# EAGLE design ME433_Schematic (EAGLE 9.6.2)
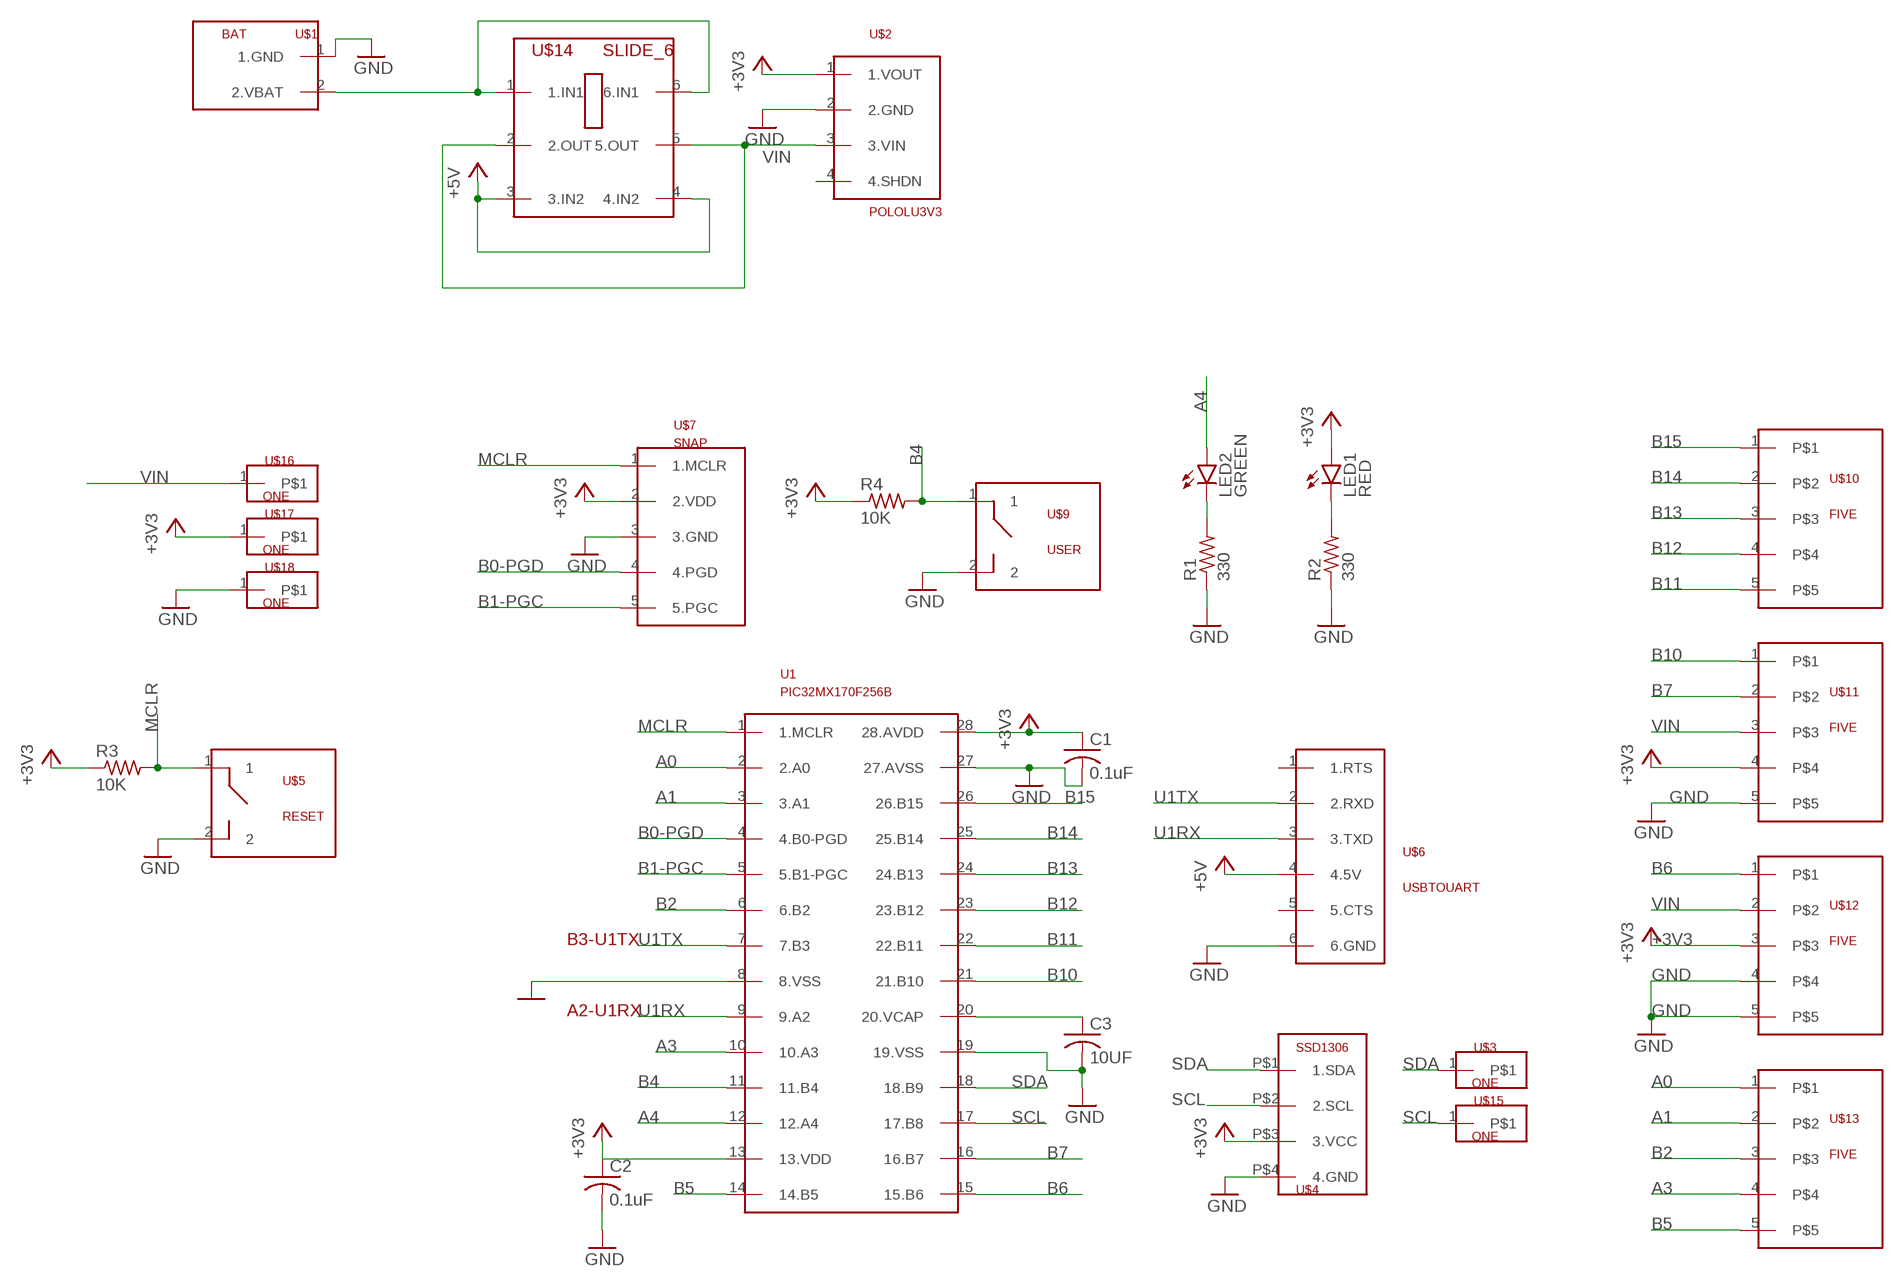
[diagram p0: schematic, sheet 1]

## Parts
C1  0.1uF  C-US025-030X050  [C025-030X050]
C2  0.1uF  C-US025-030X050  [C025-030X050]
C3  10UF  C-US025-030X050  [C025-030X050]
LED1  RED  LED3MM  [LED3MM]
LED2  GREEN  LED3MM  [LED3MM]
R1  330  R-US_0207/7  [0207/7]
R2  330  R-US_0207/7  [0207/7]
R3  10K  R-US_0207/7  [0207/7]
R4  10K  R-US_0207/7  [0207/7]
U1  PIC32MX170F256B  [DIL28-3]
U$1  BAT  [BAT]
U$2  POLOLU3V3  [POLOLU3V3]
U$3  ONE  [ONE]
U$4  SSD1306  [SSD1306]
U$5  RESET  BUTTON  [BUTTON]
U$6  USBTOUART  [USBTOUART]
U$7  SNAP  [SNAP]
U$9  USER  BUTTON  [BUTTON]
U$10  FIVE  [FIVE]
U$11  FIVE  [FIVE]
U$12  FIVE  [FIVE]
U$13  FIVE  [FIVE]
U$14  SLIDE_6  [SLIDE_6]
U$15  ONE  [ONE]
U$16  ONE  [ONE]
U$17  ONE  [ONE]
U$18  ONE  [ONE]

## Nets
+3V3: C1.1 C2.1 LED1.A R3.1 R4.1 U1.13(13.VDD) U1.28(28.AVDD) U$2.1(1.VOUT) U$4.P$3(3.VCC) U$7.2(2.VDD) U$11.4 U$12.3 U$17.1
+5V: U$6.4(4.5V) U$14.3(3.IN2) U$14.4(4.IN2)
A0: U1.2(2.A0) U$13.1
A1: U1.3(3.A1) U$13.2
A3: U1.10(10.A3) U$13.4
A4: LED2.A U1.12(12.A4)
B0-PGD: U1.4(4.B0-PGD) U$7.4(4.PGD)
B1-PGC: U1.5(5.B1-PGC) U$7.5(5.PGC)
B2: U1.6(6.B2) U$13.3
B4: R4.2 U1.11(11.B4) U$9.1
B5: U1.14(14.B5) U$13.5
B6: U1.15(15.B6) U$12.1
B7: U1.16(16.B7) U$11.2
B10: U1.21(21.B10) U$11.1
B11: U1.22(22.B11) U$10.5
B12: U1.23(23.B12) U$10.4
B13: U1.24(24.B13) U$10.3
B14: U1.25(25.B14) U$10.2
B15: U1.26(26.B15) U$10.1
GND: C1.2 C2.2 C3.2 R1.1 R2.1 U1.8(8.VSS) U1.19(19.VSS) U1.27(27.AVSS) U$1.1(1.GND) U$2.2(2.GND) U$4.P$4(4.GND) U$5.2 U$6.6(6.GND) U$7.3(3.GND) U$9.2 U$11.5 U$12.4 U$12.5 U$18.1
MCLR: R3.2 U1.1(1.MCLR) U$5.1 U$7.1(1.MCLR)
N$1: LED1.K(C) R2.2
N$2: LED2.K(C) R1.2
N$3: C3.1 U1.20(20.VCAP)
N$4: U$1.2(2.VBAT) U$14.1(1.IN1) U$14.6(6.IN1)
SCL: U1.17(17.B8) U$4.P$2(2.SCL) U$15.1
SDA: U1.18(18.B9) U$3.1 U$4.P$1(1.SDA)
U1RX: U1.9(9.A2) U$6.3(3.TXD)
U1TX: U1.7(7.B3) U$6.2(2.RXD)
VIN: U$2.3(3.VIN) U$11.3 U$12.2 U$14.2(2.OUT) U$14.5(5.OUT) U$16.1
Unconnected: U$2.4(4.SHDN) U$6.1(1.RTS) U$6.5(5.CTS)

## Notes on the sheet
- B3-U1TX
- A2-U1RX

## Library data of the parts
C1-C3 = ME433_Library:C-US: CAPACITOR, American symbol; SPICEPREFIX: C
LED1 LED2 = ME433_Library:LED: LED
R1-R4 = ME433_Library:R-US_: RESISTOR, American symbol; SPICEPREFIX: R
U1 = ME433_Library:PIC32MX170F256B
U$1 = ME433_Library:BAT
U$2 = ME433_Library:POLOLU3V3
U$3 U$15-U$18 = ME433_Library:ONE
U$4 = ME433_Library:SSD1306
U$5 U$9 = ME433_Library:BUTTON
U$6 = ME433_Library:USBTOUART
U$7 = ME433_Library:SNAP
U$10-U$13 = ME433_Library:FIVE
U$14 = ME433_Library:SLIDE_6

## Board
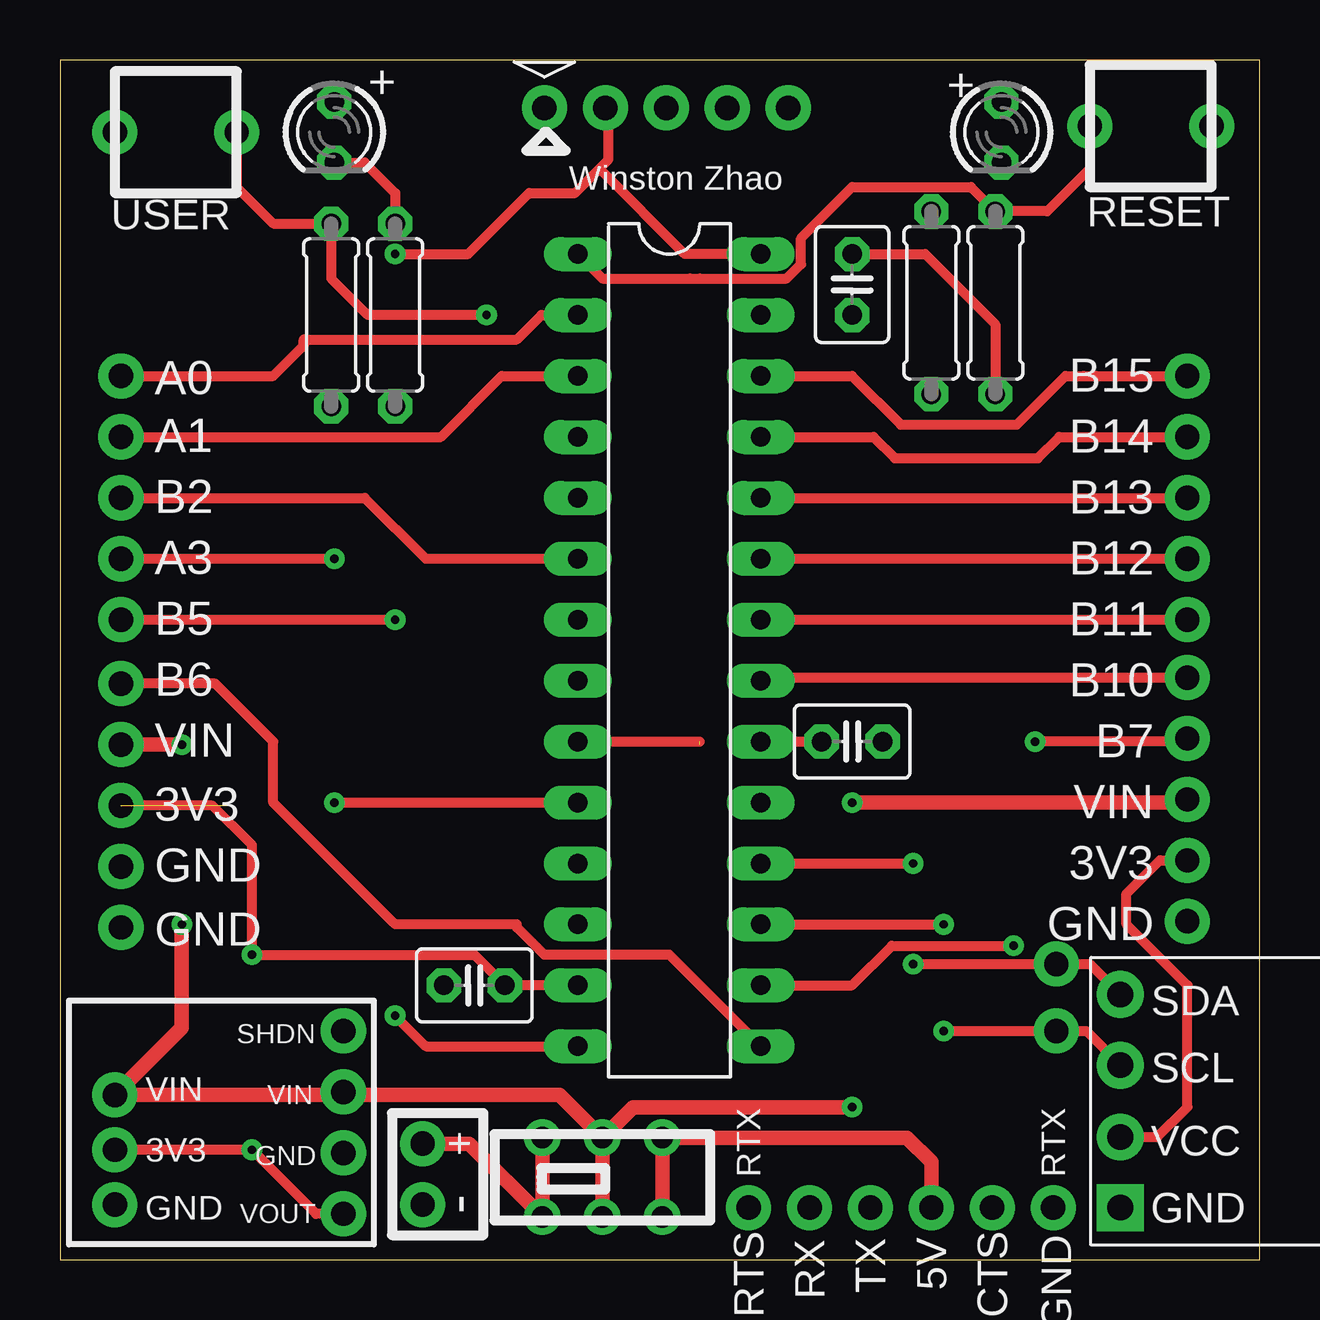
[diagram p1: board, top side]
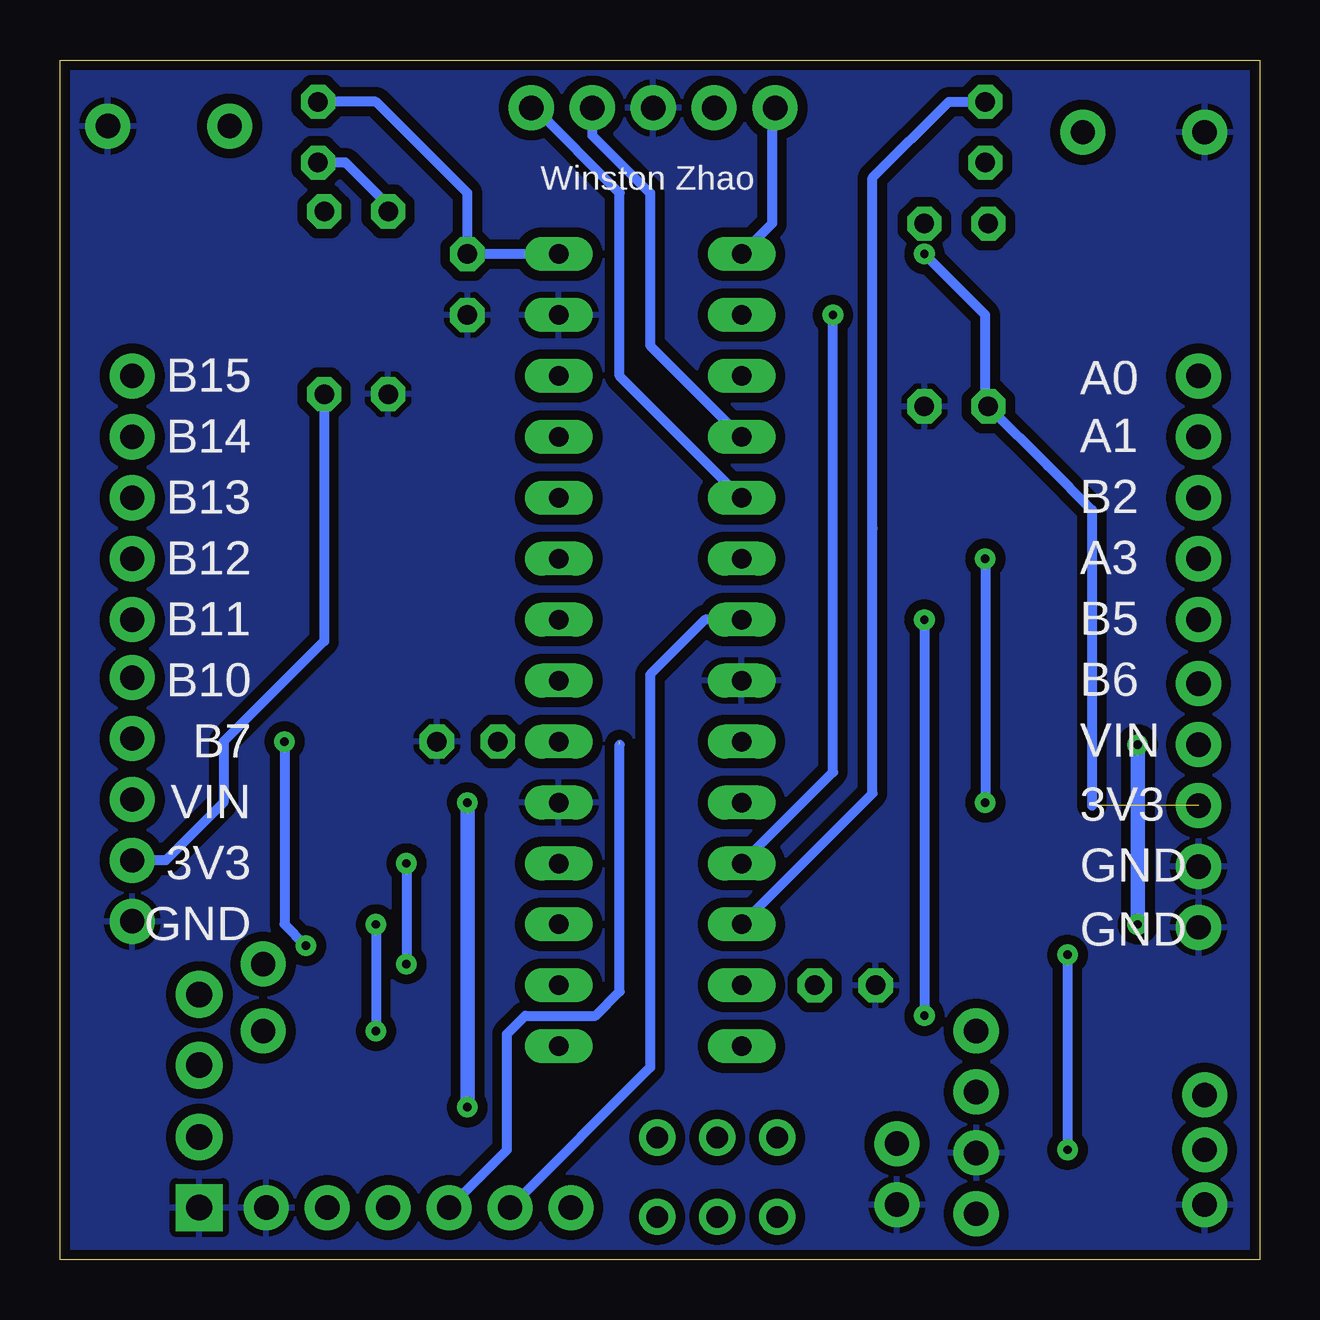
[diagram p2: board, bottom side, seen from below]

Size 50 x 50 mm. Coordinates in mm from the lower left corner, seen from the top.
Outline: 0,0 50,0 50,50 0,50 0,0
Copper layers (1*16): Top 0.035mm / dielectric 1.5mm / Bottom 0.035mm
Design rules "SparkFun": minimum track width 8mil, minimum drill 20mil, track to track 8mil, track to pad 8mil, pad to pad 8mil, via to via 8mil, smd to smd 8mil, copper to edge 8mil, drill to drill 8mil, minimum pad ring 12mil, minimum via ring 10mil, stop-mask expansion 4mil, vias tented up to drill 20mil, thermal gap 10mil

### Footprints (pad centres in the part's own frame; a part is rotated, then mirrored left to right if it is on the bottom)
C025-030X050 = drill 0.813 octagon: 1 -1.27,0; 2 1.27,0
LED3MM = drill 0.813 octagon: A -1.27,0; K 1.27,0
0207/7 = drill 0.813 octagon: 1 -3.81,0; 2 3.81,0
DIL28-3 = drill 0.813 long: 1 -16.51,-3.81; 2 -13.97,-3.81; 3 -11.43,-3.81; 4 -8.89,-3.81; 5 -6.35,-3.81; 6 -3.81,-3.81; 7 -1.27,-3.81; 8 1.27,-3.81; 9 3.81,-3.81; 10 6.35,-3.81; 11 8.89,-3.81; 12 11.43,-3.81; 13 13.97,-3.81; 14 16.51,-3.81; 15 16.51,3.81; 16 13.97,3.81; 17 11.43,3.81; 18 8.89,3.81; 19 6.35,3.81; 20 3.81,3.81; 21 1.27,3.81; 22 -1.27,3.81; 23 -3.81,3.81; 24 -6.35,3.81; 25 -8.89,3.81; 26 -11.43,3.81; 27 -13.97,3.81; 28 -16.51,3.81
BAT = drill 1.016 pad 1.88: 1 -1.27,0; 2 1.27,0
POLOLU3V3 = drill 1.016 pad 1.88: 1 0,3.81; 2 0,1.27; 3 0,-1.27; 4 0,-3.81
ONE = drill 1.016 pad 1.88: 1 0,0
SSD1306 = drill 1.067 pad 1.956: P$1 -17.78,4.445; P$2 -17.78,1.499; P$3 -17.78,-1.499 | drill 1.067 pad 1.956 square: P$4 -17.78,-4.445
BUTTON = drill 1.016 pad 1.88: 1 -2.54,0; 2 2.54,0
USBTOUART = drill 1.016 pad 1.88: 1 2.54,6.35; 2 2.54,3.81; 3 2.54,1.27; 4 2.54,-1.27; 5 2.54,-3.81; 6 2.54,-6.35
SNAP = drill 1.016 pad 1.88: 1 -5.08,0; 2 -2.54,0; 3 0,0; 4 2.54,0; 5 5.08,0
FIVE = drill 1.016 pad 1.88: 1 -5.08,0; 2 -2.54,0; 3 0,0; 4 2.54,0; 5 5.08,0
SLIDE_6 = drill 0.9: 1 -2.5,-1.65; 2 0,-1.65; 3 2.5,-1.65; 4 2.5,1.65; 5 0,1.65; 6 -2.5,1.65

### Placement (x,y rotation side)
C1  33.02,40.64 270 top
C2  17.27,11.43 180 top
C3  33.02,21.59 0 top
LED1  39.24,46.99 270 top
LED2  11.43,46.99 270 top
R1  13.97,39.37 90 top
R2  36.32,39.88 90 top
R3  38.99,39.88 90 top
R4  11.3,39.37 90 top
U1  25.4,25.4 270 top
U$1  15.11,3.56 90 top
U$2  11.81,5.71 180 top
U$3  41.53,12.32 90 top
U$4  61.98,6.6 0 top
U$5  45.47,47.24 0 top
U$6  35.05,-0.38 90 top
U$7  25.27,48.01 0 top
U$9  4.83,46.99 180 top
U$10  46.99,31.75 270 top
U$11  46.99,19.18 270 top
U$12  2.54,18.92 270 top
U$13  2.54,31.75 270 top
U$14  22.61,3.43 0 top
U$15  41.53,9.53 90 top
U$16  2.29,6.86 90 top
U$17  2.29,4.57 90 top
U$18  2.29,2.29 90 top

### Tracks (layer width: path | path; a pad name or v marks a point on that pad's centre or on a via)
+3V3  (via drill 0.35)  (1 unrouted)
  Top 0.406: U1.13 C2.1 17.27,12.7 v8,12.7 8,17.27 6.35,18.92 U$12.3 | C1.1 36.07,41.91 38.99,38.99 R3.1 | U$4.P$3 45.74,5.11 46.99,6.35 46.99,11.43 44.45,13.97 44.45,15.24 45.85,16.64 U$11.4 | U$2.1 10.67,1.91 v8,4.57 U$17.1 | v13.97,41.91 17.02,41.91 19.56,44.45 21.46,44.45 22.54,45.53 | 22.54,45.53 22.86,45.85 v22.86,47.88 | U1.28 26.04,41.91 22.54,45.4 22.54,45.53
  Bottom 0.406: LED1.A 36.83,48.26 33.02,44.45 C1.1 U1.28 | U$7.2 v22.86,47.88 | v13.97,41.91 11.43,39.37 11.43,35.69 R4.1 8.83,33.08 6.99,31.24 6.99,18.92 | R3.1 38.99,25.78 43.18,21.59 43.18,19.05 45.59,16.64 U$11.4 | v8,12.7 v8,4.57
+5V
  Top 0.61: U$14.3 U$14.4 35.31,5.08 36.32,4.06 U$6.4
A0
  Top 0.406: U$13.1 8.89,36.83 10.16,38.1 10.16,38.35 19.05,38.35 20.07,39.37 U1.2
A1
  Top 0.406: U$13.2 15.88,34.29 18.41,36.83 U1.3
A3  (via drill 0.35)
  Top 0.406: U$13.4 v11.43,29.21 | v11.43,19.05 U1.10
  Bottom 0.406: v11.43,29.21 v11.43,19.05
A4
  Bottom 0.406: LED2.A 12.95,48.26 16.13,45.09 16.13,30.48 16.13,19.43 U1.12
B0-PGD
  Bottom 0.406: U$7.4 27.81,46.86 25.4,44.45 25.4,38.1 U1.4
B1-PGC
  Bottom 0.406: U1.5 26.67,36.83 26.67,44.45 30.23,48.01 U$7.5
B2
  Top 0.406: U$13.3 12.7,31.75 15.24,29.21 U1.6
B4  (via drill 0.35)
  Top 0.406: U$9.1 7.37,44.7 8.89,43.18 R4.2 11.3,40.89 12.76,39.43 12.83,39.37 v17.78,39.37
  Bottom 0.406: U1.11 17.78,20.32 v17.78,39.37
B5  (via drill 0.35)
  Top 0.406: U$13.5 v13.97,26.67 | v13.97,10.16 15.24,8.89 U1.14
  Bottom 0.406: v13.97,26.67 v13.97,10.16
B6
  Top 0.406: U1.15 25.4,12.7 20.19,12.7 19.05,13.84 19.05,13.97 13.97,13.97 8.89,19.05 8.89,21.59 6.48,24 U$12.1
B7  (via drill 0.35)
  Top 0.406: U$11.2 46.86,21.59 v40.64,21.59 | U1.16 33.02,11.43 34.67,13.08 v39.75,13.08
  Bottom 0.406: v40.64,21.59 40.64,13.97 v39.75,13.08
B10
  Top 0.406: U1.21 29.34,24.26 U$11.1
B11
  Top 0.406: U1.22 U$10.5
B12
  Top 0.406: U1.23 U$10.4
B13
  Top 0.406: U1.24 U$10.3
B14
  Top 0.406: U$10.2 41.66,34.29 40.77,33.4 34.8,33.4 33.91,34.29 U1.25
B15
  Top 0.406: U1.26 33.02,36.83 35.05,34.8 39.88,34.8 41.91,36.83 42.67,36.83 43.18,36.83 U$10.1
GND
  pour Bottom (isolate 0.406): 0,0 50.8,0 50.8,50.8 0,50.8
MCLR
  Top 0.406: U$5.1 42.93,45.47 41.15,43.69 R3.2 37.97,44.7 33.02,44.7 30.89,42.57 30.89,41.49 30.29,40.89 26.67,40.89 26.26,40.89 22.61,40.89 U1.1
  Bottom 0.406: U$7.1 20.32,47.88 20.32,43.18 U1.1
N$1
  Bottom 0.406: LED1.K 38.1,45.72 36.32,43.94 R2.2
N$2
  Top 0.406: LED2.K 12.7,45.72 13.97,44.45 R1.2
N$3
  Top 0.406: U1.20 C3.1
N$4
  Top 0.61: U$14.6 U$14.1 17.06,4.83 U$1.2
SCL  (via drill 0.35)
  Top 0.406: U1.17 v36.83,13.97 | v36.83,9.53 U$15.1 42.77,9.53 U$4.P$2
  Bottom 0.406: v36.83,13.97 v36.83,9.53
SDA  (via drill 0.35)
  Top 0.406: U1.18 v35.56,16.51 | v35.56,12.32 U$3.1 42.93,12.32 U$4.P$1
  Bottom 0.406: v35.56,16.51 v35.56,12.32
U1RX  (1 unrouted)
  Top 0.406: U1.9 26.67,21.59
  Bottom 0.406: U$6.3 31.37,4.57 31.37,9.4 30.61,10.16 27.69,10.16 26.67,11.18 26.67,21.46
U1TX
  Bottom 0.406: U1.7 23.11,26.67 25.4,24.38 25.4,8 U$6.2
VIN  (via drill 0.35)
  Top 0.406: 11.68,6.86 U$2.3
  Top 0.61: U$14.5 U$14.2 | U$14.5 20.83,6.86 11.68,6.86 U$16.1 5.08,9.65 v5.08,13.97 | U$14.5 23.88,6.35 v33.02,6.35 | U$11.3 46.86,19.05 v33.02,19.05 | U$12.2 v5.08,21.46
  Bottom 0.61: v33.02,19.05 v33.02,6.35 | v5.08,21.46 v5.08,13.97

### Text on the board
tPlace: + | + | Winston Zhao | B15 | A0 | B14 | A1 | B13 | B2 | B12 | A3 | B11 | B5 | B10 | B6 | B7 | VIN | VIN | 3V3 | 3V3 | GND | GND | GND | VIN | 3V3 | RTX | RTX | GND
bPlace: Winston Zhao | B15 | A0 | B14 | A1 | B13 | B2 | B12 | A3 | B11 | B5 | B10 | B6 | B7 | VIN | VIN | 3V3 | 3V3 | GND | GND | GND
